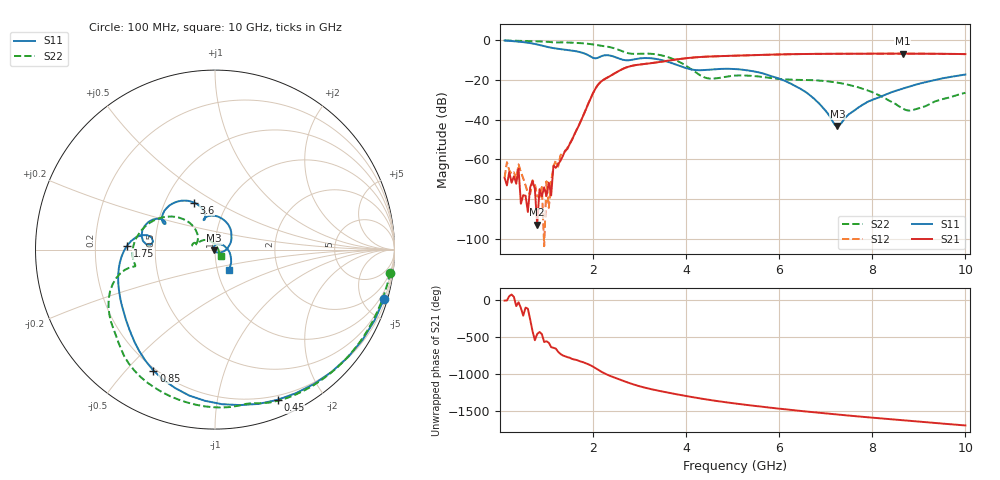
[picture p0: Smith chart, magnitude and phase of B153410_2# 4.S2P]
!  2-Port S-parameters saved by WinCal
! VAR MeasName=S-Parameters (CALIBRATED_DATA) read from VNA (N5245A)
! VAR MeasDate=2016-12-23 9:59:33
! VAR NAME=B153410_2# 4
! VAR FILENAME=B153410_2# 4.S2P
! VAR DATE=2016-12-23 9:59:33
! VAR PHYS_PORTS=1,2
# Hz S DB R 50
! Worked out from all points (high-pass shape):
!   199 points, 100 MHz to 10 GHz, reference 50 ohm
!   highest |S21| = -6.77 dB at 8.65 GHz (marker M1); lowest = -92.9 dB at 800 MHz (marker M2)
!   |S21| within 3 dB of the highest: 3.77 GHz to end of sweep
!   lowest |S11| = -43.2 dB at 7.25 GHz (marker M3), VSWR 1.01, Z = 49.4 - j0.39 ohm
!   |S11| at or under -10 dB: 2.673 GHz to 2.806 GHz (132.9 MHz wide, 4.85 % of centre); 3.471 GHz to end of sweep
!   |S22| runs from -35.4 to -0.1 dB; largest |S21 - S12| = 0.0022
!   S11 on the Smith chart (normalised r, x): 100 MHz: 0.47, -6.99; 450 MHz: 0.16, -1.49; 850 MHz: 0.19, -0.60; 1.75 GHz: 0.34, +0.02; 3.6 GHz: 0.70, +0.40; 10 GHz: 1.14, -0.26
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1e8  -0.16 -16.2  -69.35 -14.0  -69.06 105.6  -0.14 -7.5
3.5e8  -0.63 -53.4  -72.25 -87.6  -69.51 8.1  -0.31 -24.3
4e8  -0.74 -60.5  -64.69 -36.0  -62.50 135.6  -0.34 -27.6
4.5e8  -0.85 -67.4  -82.35 -113.5  -66.45 -142.6  -0.36 -30.9
6e8  -1.29 -87.4  -86.49 -122.8  -76.99 9.8  -0.45 -40.8
7e8  -1.66 -100.0  -70.82 -64.2  -70.53 125.9  -0.52 -47.4
8e8  -2.15 -111.6  -92.91 -101.3  -78.50 35.0  -0.59 -53.9
8.5e8  -2.43 -117.0  -75.01 -74.8  -79.18 -174.0  -0.63 -57.2
1e9  -3.30 -130.8  -78.36 161.1  -71.04 -156.5  -0.79 -67.1
1.05e9  -3.56 -134.7  -71.64 140.5  -84.39 -150.4  -0.87 -70.3
1.1e9  -3.79 -138.3  -78.17 82.9  -71.12 79.7  -0.98 -73.4
1.15e9  -3.99 -141.8  -63.09 73.4  -63.71 73.4  -1.10 -76.1
1.75e9  -6.19 177.4  -40.10 -112.8  -40.03 -112.2  -1.52 -113.6
2.2e9  -7.87 173.2  -20.32 104.8  -20.35 104.8  -2.88 -142.1
3.4e9  -9.63 124.4  -11.09 -141.4  -11.09 -141.6  -7.30 167.7
3.6e9  -10.84 114.1  -10.36 -166.5  -10.36 -166.6  -8.45 154.6
5.05e9  -14.53 89.7  -7.80 46.6  -7.82 46.7  -17.83 169.6
6.7e9  -28.46 -23.7  -6.91 -68.4  -6.92 -68.4  -20.11 157.0
7.25e9  -43.22 -145.2  -6.86 -101.4  -6.83 -101.4  -21.36 142.5
8.35e9  -26.83 37.3  -6.80 -162.5  -6.79 -162.4  -30.29 91.0
8.65e9  -24.40 14.8  -6.77 -178.4  -6.78 -178.4  -34.35 56.9
1e10  -17.28 -55.6  -7.02 112.1  -7.01 112.4  -26.47 -47.3
